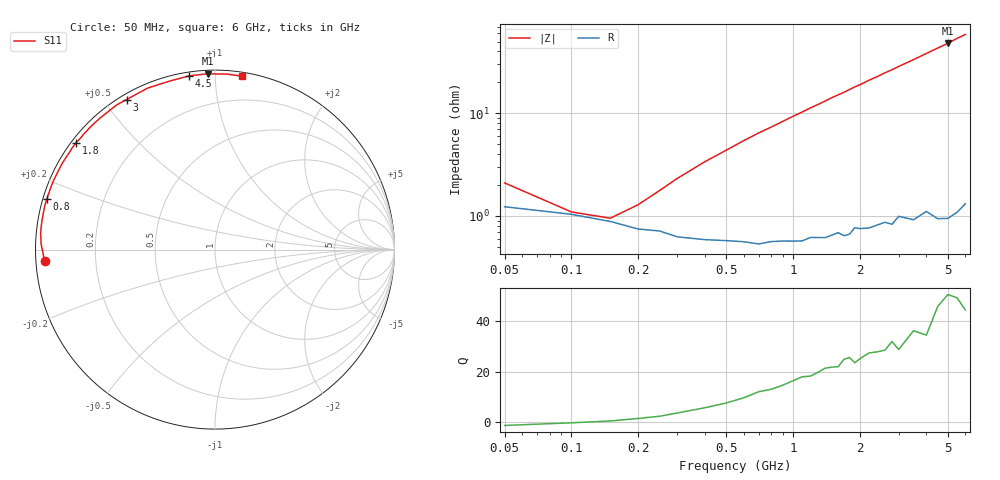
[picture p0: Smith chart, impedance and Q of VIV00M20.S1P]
! Infineon Technologies  Discrete & RF Semiconductors
! BB 804
! Si Tuning Diode in SOT23
! VR =
! S-Parameters:  July  1999
# GHz  S  MA  R  50
!  f  S11
! GHz  MAG  ANG
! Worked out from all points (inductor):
!   34 points, 50 MHz to 6 GHz, reference 50 ohm
!   read as one part to ground: L = 1.32 nH near 300 MHz
!   highest Q = 49.3 at 5 GHz (marker M1), where L = 1.53 nH
!   S11 on the Smith chart (normalised r, x): 50 MHz: 0.02, -0.03; 800 MHz: 0.01, +0.15; 1.8 GHz: 0.01, +0.34; 3 GHz: 0.02, +0.57; 4.5 GHz: 0.02, +0.86; 6 GHz: 0.03, +1.17
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0.05  0.952 -176.1
0.1  0.9593 -179.2
0.2  0.9706 177.6
0.3  0.9753 174.9
0.4  0.9768 172.4
0.5  0.9774 170.1
0.7  0.9792 165.4
0.8  0.9782 163.3
1.1  0.9783 156.8
1.2  0.9768 154.6
1.4  0.9772 150.5
1.5  0.9762 148.3
1.6  0.9751 146.4
1.7  0.977 144.5
1.8  0.9765 142.4
1.9  0.9732 140.3
2  0.974 138.6
2.2  0.9744 134.6
2.4  0.9733 131.1
2.6  0.9725 127.3
2.8  0.9744 124.1
3  0.9705 120.5
3.5  0.9749 112.7
4  0.9724 105.2
4.5  0.9787 98.4
5  0.9805 92.4
5.5  0.98 86.0
6  0.978 81.0
